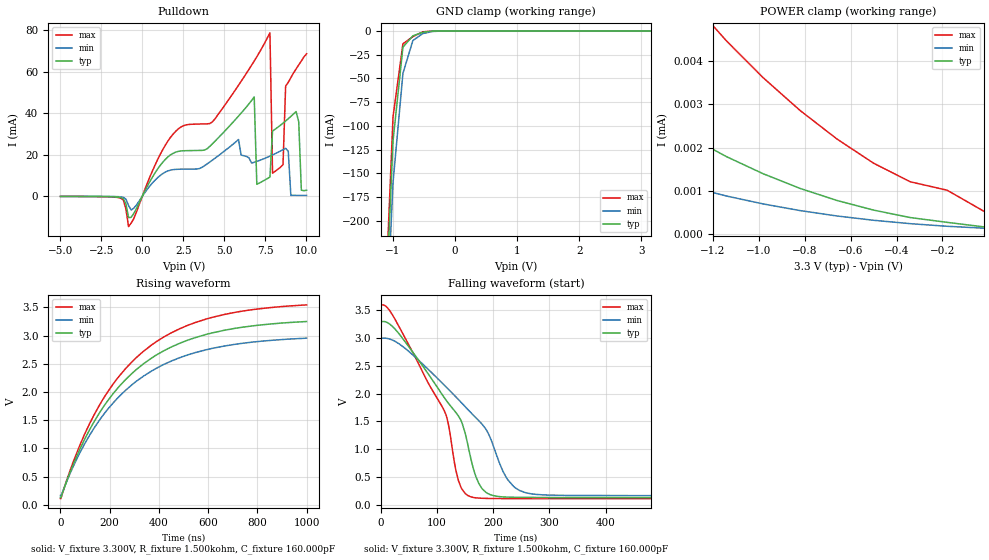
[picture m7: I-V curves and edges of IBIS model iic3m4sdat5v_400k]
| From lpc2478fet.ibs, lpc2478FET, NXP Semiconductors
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| iic3m4sdat5v
|   IIC Pad
|   5Volt tolerant
| Normal 400 kHz Open-drain Mode
[Model]   iic3m4sdat5v_400k | of iic3m4sdat5v
Model_type   I/O_open_drain
Polarity   Non-Inverting
|  Reciever Thresholds
Vinl   = 0.54V
Vinh   = 1.26V
| AC Test Load Conditions
Vref   = 1.8
Cref   = 1.6e-10
Rref   = 1500
Vmeas   = 0.9
| [Process Range]   typical   min   max
| C_comp edge width   400.000ps   400.000ps   400.000ps
| C_comp Tstrobe   40.000fs   40.000fs   40.000fs
C_comp   2.322pF   2.205pF   2.448pF
[Temperature Range]   25   125   -40
[Voltage Range]   3.30V   3.00V   3.60V
[GND Clamp Reference]   0.00V   0.00V   0.00V
[Pulldown Reference]   0.00V   0.00V   0.00V
[POWER Clamp Reference]   3.30V   3.00V   3.60V
[Pullup Reference]   3.30V   3.00V   3.60V
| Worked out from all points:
|   slope of the pulldown table from 0 to 0.495 V, typ, clamps not added: 65.7 ohm
|   GND clamp passes 1 mA (typ) near -0.48 V on its own axis
|   rising waveform, V_fixture 3.300V, R_fixture 1.500kohm, C_fixture 160.000pF: 20-80 % time 323ns typ, 323ns min, 323ns max; typ from 0.13 V to 3.25 V
|   falling waveform, V_fixture 3.300V, R_fixture 1.500kohm, C_fixture 160.000pF: 20-80 % time 98.9ns typ, 127ns min, 81.5ns max; typ from 3.3 V to 0.13 V
[GND Clamp]
| ref voltage   0.00V   0.00V   0.00V
|   Voltage   I(typ)   I(min)   I(max)
-5V       -7.859A    -7.83A     -7.884A
-1.16V    -357.8mA   -390mA     -341.6mA
-1V       -115.9mA   -159.9mA   -90.54mA
-840mV    -16.96mA   -44.54mA   -13.4mA
-680mV    -5.122mA   -10.06mA   -5.915mA
-520mV    -1.277mA   -2.664mA   -808.9uA
-360mV    -33.2uA    -452.4uA   -4.239uA
-200mV    -130.6nA   -9.498uA   -2.779nA
3.16V     74.24nA    171.4nA    36.42nA
[Power Clamp]   | Vtable = Vcc - Vpad
| ref voltage   3.30V   3.00V   3.60V
|   Voltage   I(typ)   I(min)   I(max)
-6.74V    291.1uA    143.4uA    558.6uA
-2.74V    10.23uA    5.038uA    26uA
-2.58V    8.798uA    4.367uA    21.55uA
-1.94V    4.749uA    2.342uA    10.7uA
-1.62V    3.353uA    1.636uA    7.693uA
-1.3V     2.244uA    1.093uA    5.416uA
-1.14V    1.786uA    876.4nA    4.461uA
-820mV    1.053uA    540.3nA    2.856uA
-500mV    551.5nA    316.1nA    1.637uA
-340mV    378.8nA    237.6nA    1.207uA
-180mV    268.4nA    177.3nA    1.013uA
-20mV     163.8nA    133.4nA    527nA
[Pulldown]
| ref voltage   0.00V   0.00V   0.00V
|   Voltage   I(typ)   I(min)   I(max)
-5V       -38.11uA   -18.94uA   -68.97uA
-840mV    -10.24mA   -4.401mA   -14.56mA
1.72V     19.93mA    12.59mA    28.35mA
6.84V     47.86mA    16.41mA    65.1mA
7V        5.817mA    16.83mA    67.16mA
7.8V      9.294mA    19.34mA    78.67mA
7.96V     31.39mA    19.92mA    11.11mA
8.6V      35.21mA    22.46mA    15.25mA
8.76V     36.26mA    23.1mA     53.01mA
9.4V      40.79mA    465uA      61.3mA
9.72V     2.965mA    445.7uA    65.13mA
10.04V    2.979mA    443.5uA    68.57mA
[Ramp]
R_load   = 90.000ohm
|   dV/dt(typ)   dV/dt(min)   dV/dt(max)
dV/dt_r   601.136mV/250.000ps   360.347mV/300.000ps   884.382mV/200.000ps
dV/dt_f   600.945mV/151.250ns   360.044mV/164.150ns   884.281mV/126.000ns
[Rising Waveform]  | cubic spline decimation from 20001 points
V_fixture   = 3.300V
V_fixture_min = 3.000V
V_fixture_max = 3.600V
R_fixture   = 1.500kohm
C_fixture   = 160.000pF
|   Time   V(typ)   V(min)   V(max)
0s        129.8mV    164.8mV    109.9mV
76.65ns   964.5mV    903.7mV    1.035V
118.8ns   1.335V     1.236V     1.443V
154.9ns   1.605V     1.478V     1.739V
241.1ns   2.11V      1.931V     2.293V
336.9ns   2.498V     2.279V     2.719V
447.9ns   2.792V     2.543V     3.042V
593.4ns   3.021V     2.749V     3.294V
782.8ns   3.172V     2.885V     3.46V
1us       3.248V     2.953V     3.542V
[Falling Waveform]  | cubic spline decimation from 20001 points
V_fixture   = 3.300V
V_fixture_min = 3.000V
V_fixture_max = 3.600V
R_fixture   = 1.500kohm
C_fixture   = 160.000pF
|   Time   V(typ)   V(min)   V(max)
0s        3.3V       3V         3.599V
32ns      3.089V     2.904V     3.223V
113.8ns   1.922V     2.149V     1.682V
138.1ns   1.604V     1.899V     449.9mV
158.9ns   901.7mV    1.676V     149.5mV
169.5ns   505.7mV    1.567V     125.4mV
186.9ns   227.2mV    1.367V     115.3mV
226ns     138.4mV    452.9mV    111.7mV
264.9ns   132.7mV    202.7mV    110.7mV
1us       129.8mV    164.8mV    109.9mV
